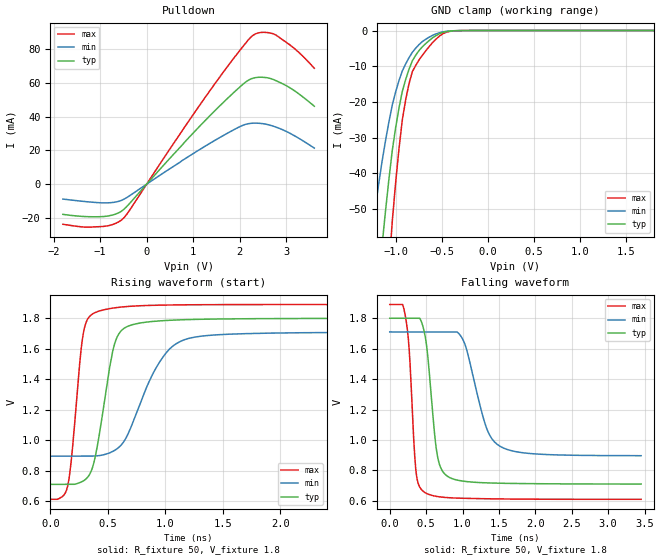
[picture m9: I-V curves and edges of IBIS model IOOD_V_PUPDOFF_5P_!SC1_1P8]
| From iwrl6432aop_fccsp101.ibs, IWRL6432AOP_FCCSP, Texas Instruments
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|   Model Cell IOOD_V_PUPDOFF_5P_!SC1_1P8
|IOOD_V_PUPDOFF_5P_!SC1_1P8
[Model]   IOOD_V_PUPDOFF_5P_!SC1_1P8
Model_type   I/O_open_drain
Polarity   Non-Inverting
Enable   Active-Low
Vinl =  0.63
Vinh =  1.17
Cref =  15pF
Rref =  100.0000M
Vref =  0V
Vmeas =  0.9
|   typ   min   max
C_comp   2.233931p   2.204415p   2.290246p
[Model Spec]
Vinl   0.63   0.5985   0.6615
Vinh   1.17   1.1115   1.2285
[Temperature Range]   25   125   -40
[Voltage Range]   1.8   1.71   1.89
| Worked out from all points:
|   slope of the pulldown table from 0 to 0.27 V, typ, clamps not added: 32.2 ohm
|   GND clamp passes 1 mA (typ) near -0.53 V on its own axis
|   rising waveform, R_fixture 50, V_fixture 1.8: 20-80 % time 141ps typ, 294ps min, 91.6ps max; typ from 0.709 V to 1.8 V
|   falling waveform, R_fixture 50, V_fixture 1.8: 20-80 % time 128ps typ, 263ps min, 86.3ps max; typ from 1.8 V to 0.71 V
| Where Nom  PVT is Nominal Process, 1.8V, 25C
|   Fast PVT is Strong Process,  1.89V, -40C
|   Slow PVT is Weak Process,   1.71V, 125C
[Pulldown]
|   voltage   I(typ)   I(min)   I(max)
-1.8V     -17.92mA   -8.85mA    -23.8mA
-1.309V   -19.26mA   -10.37mA   -25.5mA
-927.3mV  -19.22mA   -11.12mA   -25.08mA
-654.5mV  -17.65mA   -10.56mA   -23.13mA
-490.9mV  -14.97mA   -8.985mA   -20.05mA
1.364V    40.78mA    24.32mA    55.7mA
2.073V    59.41mA    35mA       81.91mA
2.291V    62.96mA    36.2mA     88.48mA
2.509V    63.41mA    35.84mA    90.12mA
2.782V    61.38mA    33.82mA    88.42mA
3.218V    54.59mA    28.02mA    79.45mA
3.6V      46.26mA    21.39mA    68.79mA
[GND_clamp]
|   voltage   I(typ)   I(min)   I(max)
-1.8V     -270.2mA   -170.2mA   -430.1mA
-1.255V   -91.66mA   -55.91mA   -148.4mA
-1.145V   -59.91mA   -36.45mA   -97.09mA
-1.109V   -50.48mA   -30.83mA   -81.55mA
-1.073V   -41.73mA   -25.65mA   -67.05mA
-1.036V   -33.66mA   -20.92mA   -53.59mA
-927.3mV  -17.07mA   -11.35mA   -25.04mA
-854.5mV  -10.86mA   -7.617mA   -14.91mA
-781.8mV  -6.919mA   -4.945mA   -9.771mA
-636.4mV  -2.823mA   -1.868mA   -4.529mA
-381.8mV  -84.73uA   -78.82uA   -126.1uA
1.8V      19.3nA     350.9nA    215.8nA
[Ramp]
| variable   typ   min   max
dV/dt_f 0.66582249/0.13069096n 0.49991745/0.26945059n 0.77756876/87.983914p
dV/dt_r 0.66457062/0.17691361n 0.50985211/0.36481894n   0.781455/0.10527652n
R_load = 50
[Rising Waveform]
R_fixture = 50
V_fixture = 1.8
V_fixture_min = 1.71
V_fixture_max = 1.89
|   time   V(typ)   V(min)   V(max)
0s        709.3mV    894.4mV    611.2mV
149.8ps   709.3mV    894.4mV    694.5mV
187.6ps   709.3mV    894.4mV    904mV
280.8ps   729.4mV    894.4mV    1.671V
386.4ps   875.3mV    895.7mV    1.836V
549.1ps   1.604V     928.2mV    1.867V
678.4ps   1.748V     1.045V     1.877V
932.6ps   1.781V     1.491V     1.885V
1.179ns   1.791V     1.662V     1.888V
3.453ns   1.8V       1.708V     1.89V
[Falling Waveform]
R_fixture = 50
V_fixture = 1.8
V_fixture_min = 1.71
V_fixture_max = 1.89
|   time   V(typ)   V(min)   V(max)
0s        1.8V       1.71V      1.89V
215.1ps   1.8V       1.71V      1.814V
269.6ps   1.8V       1.71V      1.578V
357.6ps   1.8V       1.71V      808.4mV
465ps     1.73V      1.71V      660.9mV
646.5ps   919.6mV    1.71V      629mV
789ps     762.9mV    1.71V      621.3mV
1.018ns   728.9mV    1.647V     616.7mV
1.502ns   715.8mV    962.5mV    612.4mV
3.453ns   710.3mV    896.7mV    610mV
